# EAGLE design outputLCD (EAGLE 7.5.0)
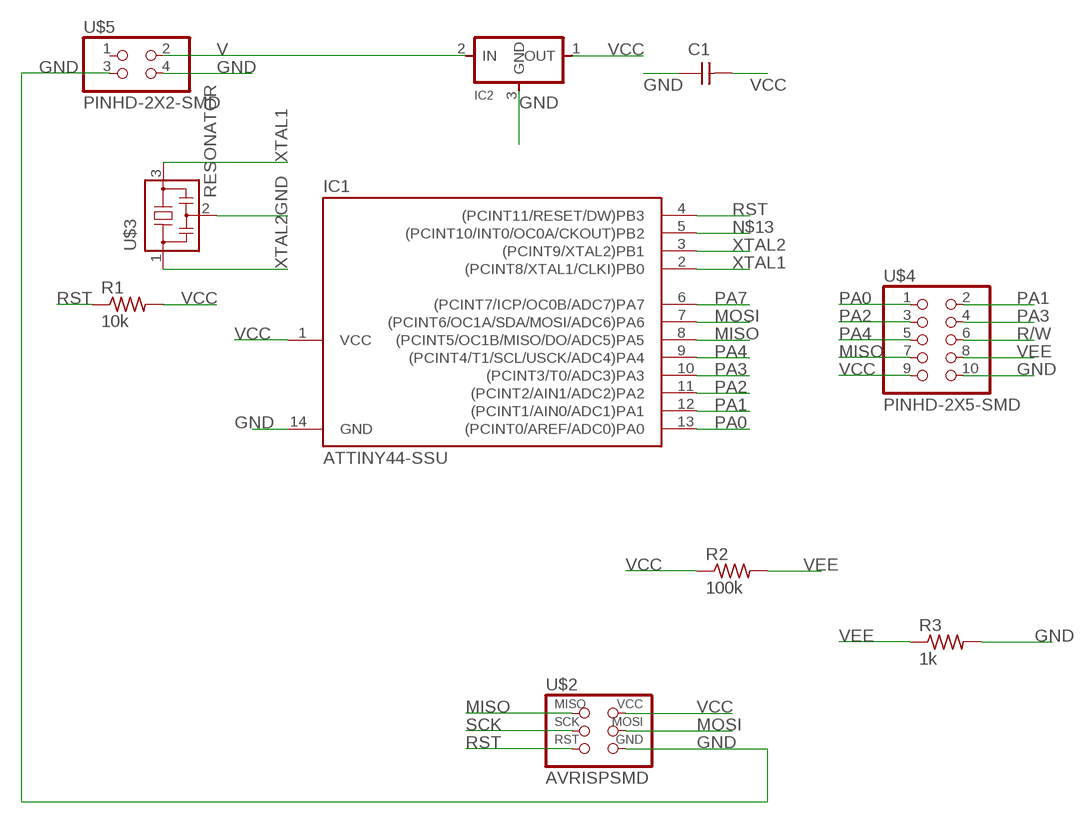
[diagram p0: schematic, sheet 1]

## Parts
C1  CAP-UNPOLARIZEDFAB  [C1206FAB]
IC1  ATTINY44-SSU  [SOIC14]
IC2  REGULATORSOT23  [SOT23]
R1  10k  RES-US1206FAB  [R1206FAB]
R2  100k  RES-US1206FAB  [R1206FAB]
R3  1k  RES-US1206FAB  [R1206FAB]
U$2  AVRISPSMD  [2X03SMD]
U$3  RESONATOR  [EFOBM]
U$4  PINHD-2X5-SMD  [2X05SMD]
U$5  PINHD-2X2-SMD  [2X02SMD]

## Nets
GND: C1.1 IC1.14(GND) IC2.3(GND) R3.2 U$2.6(GND) U$3.2 U$4.10 U$5.3 U$5.4
MISO: IC1.8((PCINT5/OC1B/MISO/DO/ADC5)PA5) U$2.1(MISO) U$4.7
MOSI: IC1.7((PCINT6/OC1A/SDA/MOSI/ADC6)PA6) U$2.4(MOSI)
N$13: IC1.5((PCINT10/INT0/OC0A/CKOUT)PB2)
PA0: IC1.13((PCINT0/AREF/ADC0)PA0) U$4.1
PA1: IC1.12((PCINT1/AIN0/ADC1)PA1) U$4.2
PA2: IC1.11((PCINT2/AIN1/ADC2)PA2) U$4.3
PA3: IC1.10((PCINT3/T0/ADC3)PA3) U$4.4
PA4: IC1.9((PCINT4/T1/SCL/USCK/ADC4)PA4) U$4.5
PA7: IC1.6((PCINT7/ICP/OC0B/ADC7)PA7)
R/W: U$4.6
RST: IC1.4((PCINT11/RESET/DW)PB3) R1.1 U$2.5(RST)
SCK: U$2.3(SCK)
V: IC2.2(IN) U$5.2
VCC: C1.2 IC1.1(VCC) IC2.1(OUT) R1.2 R2.1 U$2.2(VCC) U$4.9
VEE: R2.2 R3.1 U$4.8
XTAL1: IC1.2((PCINT8/XTAL1/CLKI)PB0) U$3.3
XTAL2: IC1.3((PCINT9/XTAL2)PB1) U$3.1
Unconnected: U$5.1

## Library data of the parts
C1 = fab:CAP-UNPOLARIZED
IC1 = fab:ATTINY44
IC2 = fab:REGULATOR
R1-R3 = fab:RES-US: Resistor (US Symbol)
U$2 = fab:AVRISP
U$3 = fab:RESONATOR
U$4 = fab:PINHD-2X5-SMD
U$5 = fab:PINHD-2X2-SMD

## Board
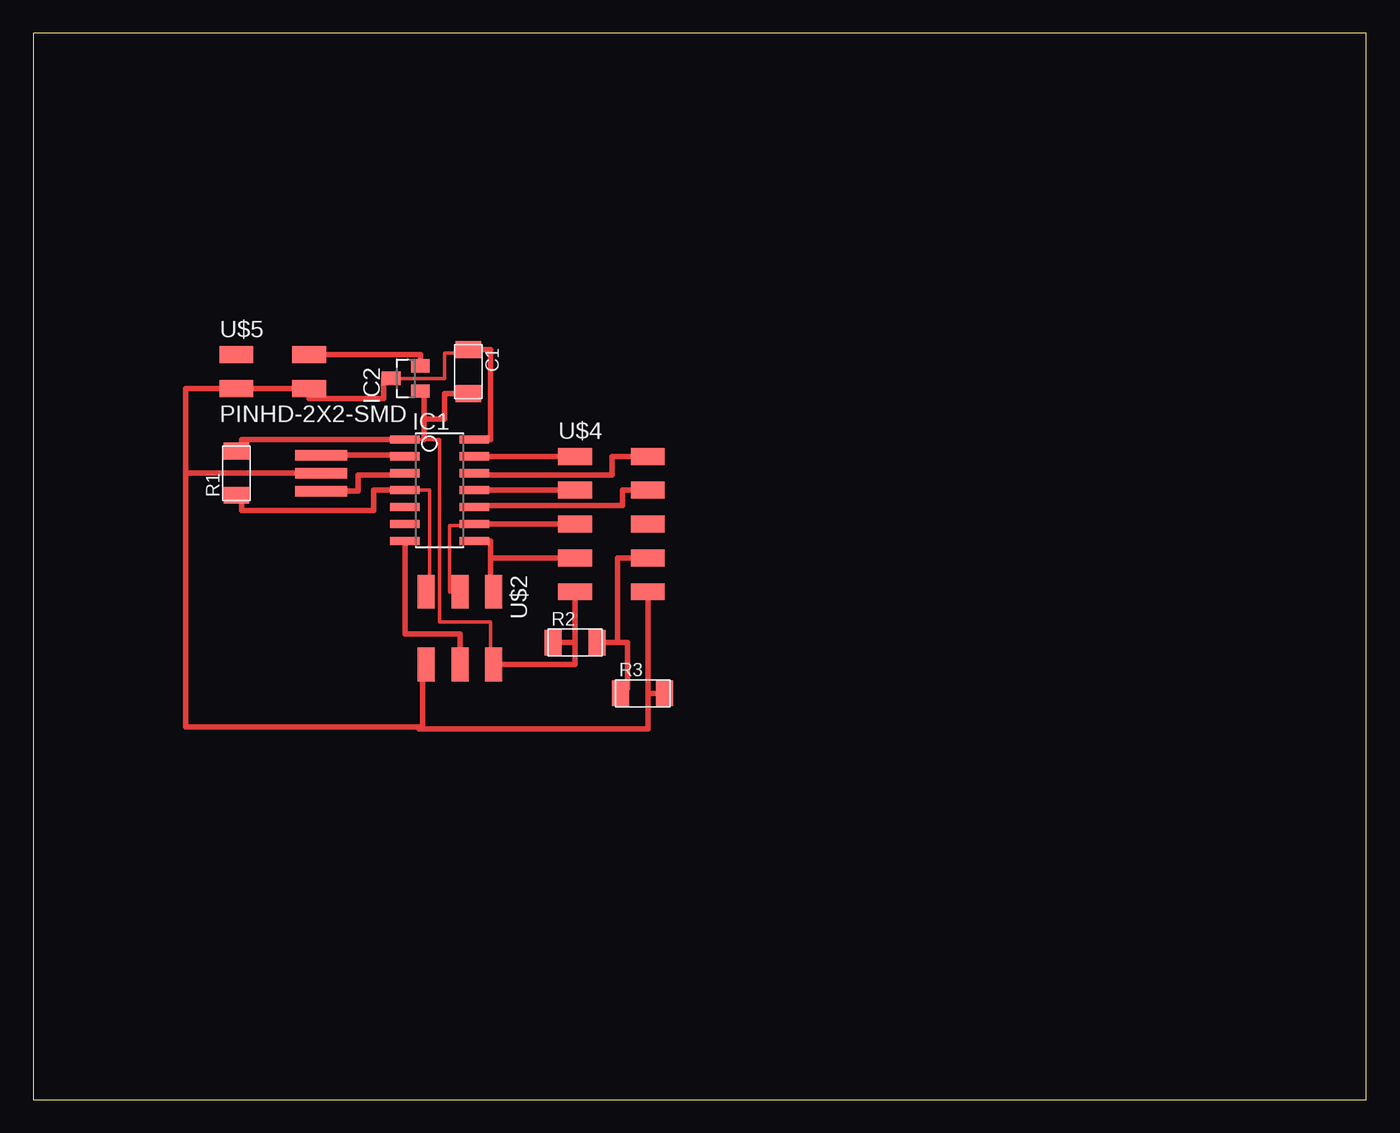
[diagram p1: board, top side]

Size 100 x 80 mm. Coordinates in mm from the lower left corner, seen from the top.
Outline: 0,0 100,0 100,80 0,80 0,0
Copper layers (1*16): Top 0.035mm / dielectric 1.5mm / Bottom 0.035mm
Design rules "default": minimum track width 10mil, minimum drill 24mil, track to track 8mil, track to pad 8mil, pad to pad 8mil, via to via 8mil, smd to smd 8mil, copper to edge 40mil, drill to drill 8mil, minimum pad ring 10mil, minimum via ring 8mil, stop-mask expansion 4mil, vias tented up to drill 0mil, thermal gap 10mil

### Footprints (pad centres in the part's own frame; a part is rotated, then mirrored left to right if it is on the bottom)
C1206FAB = smd 1.27 x 1.905: 1 -1.651,0; 2 1.651,0
SOIC14 = smd 0.61 x 2.21: 1 -3.81,-2.603; 2 -2.54,-2.603; 3 -1.27,-2.603; 4 0,-2.603; 5 1.27,-2.603; 6 2.54,-2.603; 7 3.81,-2.603; 8 3.81,2.603; 9 2.54,2.603; 10 1.27,2.603; 11 0,2.603; 12 -1.27,2.603; 13 -2.54,2.603; 14 -3.81,2.603
SOT23 = smd 1 x 1.4: 1 -0.95,-1.1; 2 0.95,-1.1; 3 0,1.1
R1206FAB = smd 1.27 x 1.905: 1 -1.651,0; 2 1.651,0
2X03SMD = smd 2.54 x 1.27: 1 -2.54,2.54; 2 2.92,2.54; 3 -2.54,0; 4 2.92,0; 5 -2.54,-2.54; 6 2.92,-2.54
EFOBM = smd 0.8 x 3.9: 1 -1.35,0; 2 0,0; 3 1.35,0
2X05SMD = smd 2.54 x 1.27: 1 -2.54,2.54; 2 2.92,2.54; 3 -2.54,0; 4 2.92,0; 5 -2.54,-2.54; 6 2.92,-2.54; 7 -2.54,-5.08; 8 2.92,-5.08; 9 -2.54,-7.62; 10 2.92,-7.62
2X02SMD = smd 2.54 x 1.27: 1 -2.54,1.27; 2 2.92,1.27; 3 -2.54,-1.27; 4 2.92,-1.27

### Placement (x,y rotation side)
C1  32.64,54.61 270 top
IC1  30.48,45.72 270 top
IC2  27.94,54.1 90 top
R1  15.24,46.99 90 top
R2  40.64,34.29 0 top
R3  45.72,30.48 0 top
U$2  32,35.56 270 top
U$3  21.59,46.99 90 top
U$4  43.18,45.72 0 top
U$5  17.78,54.61 0 top

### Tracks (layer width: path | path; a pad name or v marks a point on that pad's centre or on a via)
GND
  Top 0.254: IC2.3 30.86,54.1 30.86,56.01 33.15,56.01 33.15,56.26
  Top 0.406: C1.1 33.15,56.26 34.29,56.26 34.29,49.53 IC1.14 | IC2.3 26.29,54.1 26.29,52.58 20.7,52.58 U$5.4 U$5.3 11.43,53.34 11.43,46.99 | U$2.6 29.21,32.64 29.21,27.94 28.96,27.94 | 28.96,27.94 11.43,27.94 11.43,46.99 | U$4.10 46.1,30.48 | 46.1,30.48 46.1,27.81 28.96,27.81 28.96,27.94 | R3.2 46.1,30.48 | U$3.2 11.43,46.99
MISO
  Top 0.406: U$2.1 34.29,38.1 34.29,40.64 | IC1.8 34.29,41.91 34.29,40.64 | U$4.7 34.29,40.64
MOSI
  Top 0.406: U$2.4 32,34.92 27.88,34.92 IC1.7
PA0
  Top 0.406: U$4.1 IC1.13
PA1
  Top 0.406: U$4.2 43.43,48.26 43.43,46.86 33.08,46.86 IC1.12
PA2
  Top 0.406: U$4.3 IC1.11
PA3
  Top 0.406: U$4.4 44.2,45.72 44.2,44.58 33.08,44.58 IC1.10
PA4
  Top 0.406: U$4.5 IC1.9
RST
  Top 0.254: U$2.5 29.72,38.1 29.72,45.72 IC1.4
  Top 0.406: R1.1 15.62,45.34 15.62,44.2 25.53,44.2 25.53,45.72 IC1.4
SCK
  Top 0.254: U$2.3 31.24,38.1 31.24,43.05 33.08,43.05
V
  Top 0.406: U$5.2 29.04,55.88 IC2.2
VCC
  Top 0.254: U$2.2 34.29,32.64 34.29,35.81 30.48,35.81 30.48,49.53 29.34,49.53 IC1.1
  Top 0.406: IC2.1 29.34,53.15 29.34,51.05 | 29.34,51.05 29.34,49.53 | C1.2 30.86,52.96 30.86,51.05 29.34,51.05 | U$4.9 40.64,34.29 | 40.64,34.29 R2.1 | U$2.2 40.64,32.64 40.64,34.29 | R1.2 15.62,48.64 15.62,49.53 IC1.1
VEE
  Top 0.406: U$4.8 43.81,40.64 43.81,34.29 R2.2 44.58,34.29 44.58,30.86 44.07,30.86 R3.1
XTAL1
  Top 0.406: U$3.3 27.88,48.34 IC1.2
XTAL2
  Top 0.406: U$3.1 24.38,45.64 24.38,46.86 27.88,46.86 IC1.3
